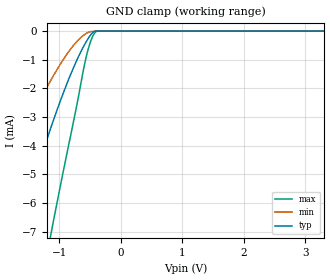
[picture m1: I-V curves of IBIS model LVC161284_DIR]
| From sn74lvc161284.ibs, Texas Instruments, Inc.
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[Model]   LVC161284_DIR
Model_type  Input
Vinl=0.8
Vinh=2.0
| variable   typ   min   max
C_comp   1.16pF   0.74pF   1.36pF
[Temperature Range]   40   100   -40
| Ambient temperature   25   85   -40
[Voltage range]   3.3   3   3.6
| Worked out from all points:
|   GND clamp passes 1 mA (typ) near -0.71 V on its own axis
[GND Clamp]
| LVC161284_DIR
|   Voltage   I(typ)   I(min)   I(max)
-5.5V     -38.52mA   -24.66mA   -66.57mA
-2.3V     -11.74mA   -7.062mA   -21.51mA
-2.22V    -11.12mA   -6.656mA   -20.45mA
-1.72V    -7.338mA   -4.213mA   -14.01mA
-1.655V   -6.866mA   -3.91mA    -13.2mA
-1.38V    -4.936mA   -2.685mA   -9.858mA
-1.13V    -3.303mA   -1.673mA   -6.976mA
-845mV    -1.65mA    -702.3uA   -3.914mA
-580mV    -426uA     -102.5uA   -1.042mA
-490mV    -124.6uA   -17.86uA   -339.5uA
-405mV    -112.8nA   -5.339uA   -20.87uA
3.3V      12.33pA    77.49pA    9.9pA
